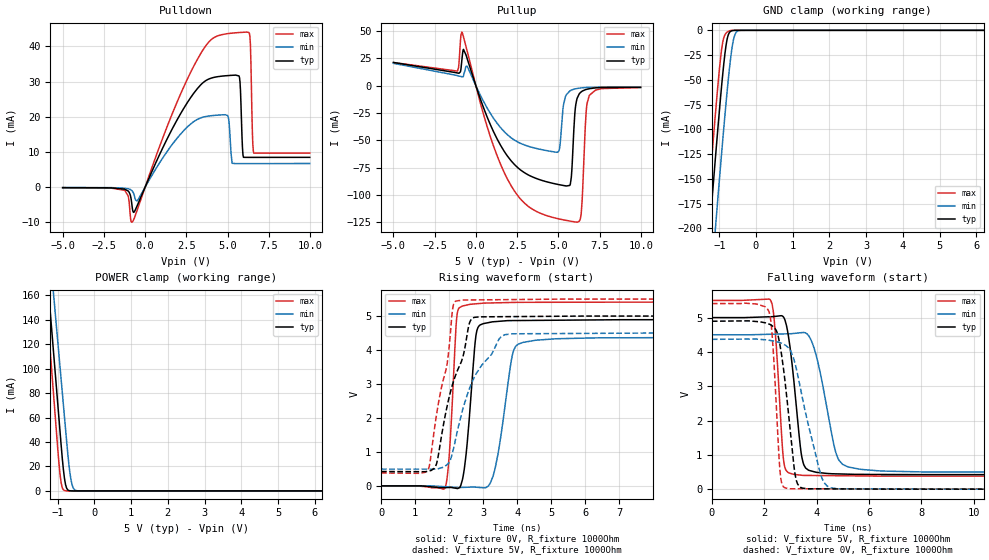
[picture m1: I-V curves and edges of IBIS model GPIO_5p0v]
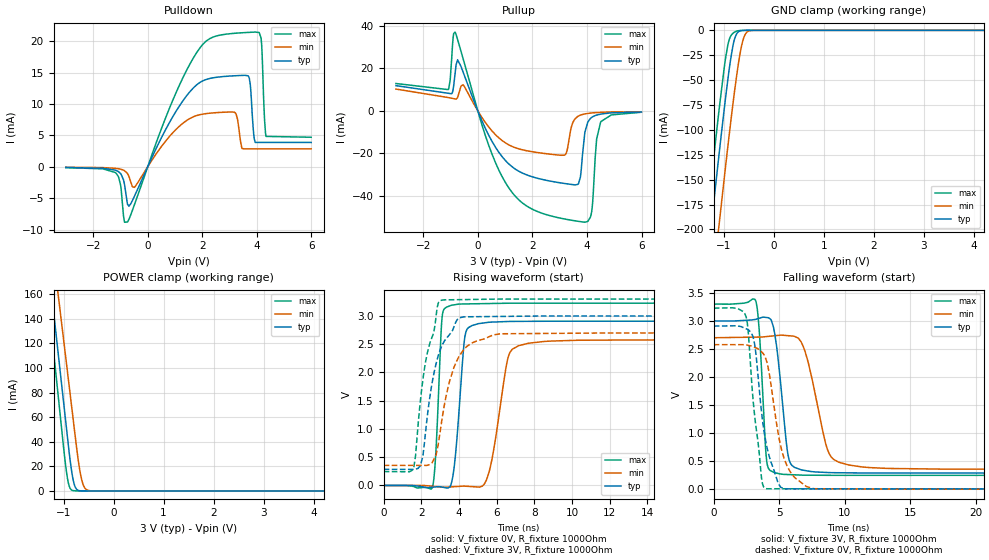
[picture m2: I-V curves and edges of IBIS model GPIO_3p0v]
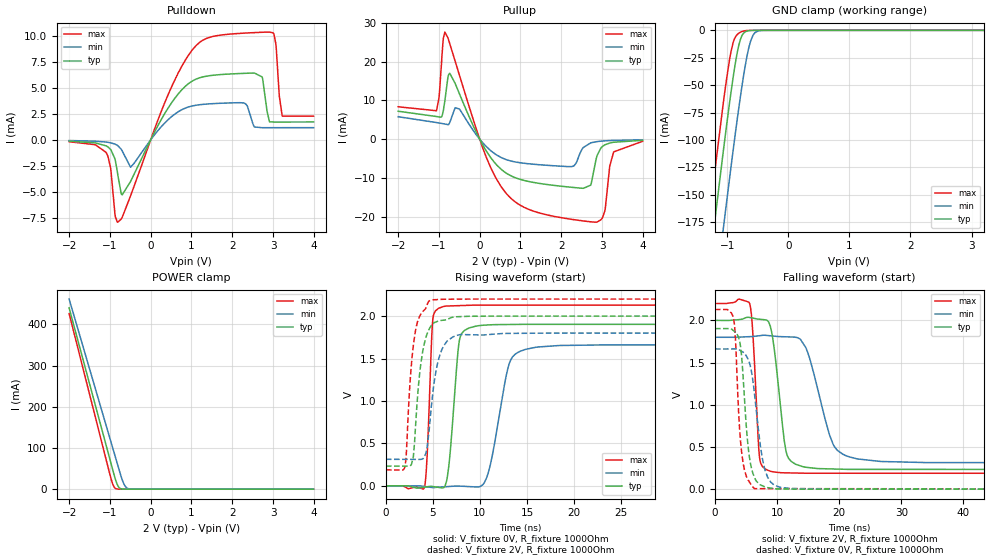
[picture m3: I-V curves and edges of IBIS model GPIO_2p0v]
|Texas Instruments Incorporated
| LMP92018: Analog System Monitor and Controller
| Marketing part#   Digital Voltage Range   Package-type   #pins
| LMP92018   1.8 to 5.5 V   LLP36   36
[IBIS Ver]   4.0
[File name]   lmp92018.ibs
[File Rev]   1.0
[Date]   02/22/2012
[Source]   Texas Instruments Incorporated.
   Analog-eLab, HPA
   12500 TI Blvd
   Dallas, TX -75243
   For Support e-mail: elab_ibis@list.ti.com
[Notes]   Revision History:
   1.0: 02/22/2012
   - Initial version of the model
   - Initial Model generated from simulations
   - Model not matched to measurements
   - Models with trailing _5p0v are generated based on 5.0V
   power supply.
   - Models with trailing _3p0v are generated based on 3.0V
   power supply.
   - Models with trailing _2p0v are generated based on 2.0V
   power supply.
   - C_comp although listed in numerical order of value are
   obtained from varying PVT conditions. For PVT conditions
   for each specific value refer the buffer description under
   respective [Model]. IBIS model user is responsible for using
   appropriate C_comp to simulate for Signal Integrity.
   - Combined pullup/Pulldown non-monotonic warning for DOUT_xxxx and GPIO_xxxx ,is based on
   SPICE simulations and accepted.
[Disclaimer]
  This model is designed as an aid for customers of Texas Instruments.
  TI and its licensors and suppliers make no warranties, either expressed
  or implied, with respect to this model, including the warranties of
  merchantability or fitness for a particular purpose.  The model is
  provided solely on an "as is" basis.  The entire risk as to its quality
  and performance is with the customer.
[Copyright] (C) Copyright 2012 Texas Instruments Incorporated.
   All rights reserved.
|   Device
[Component]   LMP92018
[Manufacturer] TI
[Package]   | 36 pin LLP
| variable   typ   min   max
R_pkg   0.01   0.008   0.12
L_pkg   0.1nH   0.08nH   0.12nH
C_pkg   0.1pF   0.08pF   0.12pF
|-------------------------PIN------------------------------------------------
[Pin] signal_name  model_name  R_pin  L_pin C_pin
1   VDD   POWER   NA   NA   NA
2   GND   GND   NA   NA   NA
3   GND   GND   NA   NA   NA
4   VGPIO   POWER   NA   NA   NA
5   VIO   POWER   NA   NA   NA
6   CSB   DIN   NA   NA   NA
7   SCLK   DIN   NA   NA   NA
8   DIN   DIN   NA   NA   NA
9   DOUT   DOUT   NA   NA   NA
10   OUT3   TERM   NA   NA   NA
11   OUT2   TERM   NA   NA   NA
12   OUT1   TERM   NA   NA   NA
13   OUT0   TERM   NA   NA   NA
14   GND   GND   NA   NA   NA
15   GPIO11   GPIO   NA   NA   NA
16   GPIO10   GPIO   NA   NA   NA
17   GPIO9   GPIO   NA   NA   NA
18   GPIO8   GPIO   NA   NA   NA
19   DRDYB   GPIO   NA   NA   NA
20   GPIO7   GPIO   NA   NA   NA
21   GPIO6   GPIO   NA   NA   NA
22   GPIO5   GPIO   NA   NA   NA
23   GPIO4   GPIO   NA   NA   NA
24   GPIO3   GPIO   NA   NA   NA
25   GPIO2   GPIO   NA   NA   NA
26   GPIO1   GPIO   NA   NA   NA
27   GPIO0   GPIO   NA   NA   NA
28   IN0   TERM   NA   NA   NA
29   IN1   TERM   NA   NA   NA
30   IN2   TERM   NA   NA   NA
31   IN3   TERM   NA   NA   NA
32   IN4   TERM   NA   NA   NA
33   IN5   TERM   NA   NA   NA
34   IN6   TERM   NA   NA   NA
35   IN7   TERM   NA   NA   NA
36   REF   TERM   NA   NA   NA
[Model Selector] GPIO
GPIO_5p0v   model for 5.0v operation
GPIO_3p0v   model for 3.0v operation
GPIO_2p0v   model for 2.0v operation
[Model Selector] DRDYB
DRDYB_5p0v   model for 5.0v operation
DRDYB_3p0v   model for 3.0v operation
DRDYB_2p0v   model for 2.0v operation
[Model Selector] DOUT
DOUT_5p0v   model for 5.0v operation
DOUT_3p0v   model for 3.0v operation
DOUT_2p0v   model for 2.0v operation
[Model Selector] DIN
DIN_5p0v   model for 5.0v operation
DIN_3p0v   model for 3.0v operation
DIN_2p0v   model for 2.0v operation
[Model Selector] TERM
TERM_5p0v   model for 5.0v operation
TERM_3p0v   model for 3.0v operation
TERM_2p0v   model for 2.0v operation
|   Model
[Model] TERM_5p0v
Model_type Terminator
C_comp   1fF   1fF   1fF
| variable   typ   min   max
[Voltage Range]   5.0V   4.5V   5.5V
[POWER Clamp Reference]  3.3V   3.0V   3.6V
[GND Clamp Reference]   0.0V   0.0V   0.0V
|Operating Temperature
[Temperature Range]   27   125   -40
|   Model
[Model] TERM_3p0v
Model_type Terminator
C_comp   1fF   1fF   1fF
| variable   typ   min   max
[Voltage Range]   3.0V   2.7V   3.3V
[POWER Clamp Reference]  3.3V   3.0V   3.6V
[GND Clamp Reference]   0.0V   0.0V   0.0V
|Operating Temperature
[Temperature Range]   27   125   -40
|   Model
[Model] TERM_2p0v
Model_type Terminator
C_comp   1fF   1fF   1fF
| variable   typ   min   max
[Voltage Range]   2.0V   1.8V   2.2V
[POWER Clamp Reference]  2.0V   1.8V   2.2V
[GND Clamp Reference]   0.0V   0.0V   0.0V
|Operating Temperature
[Temperature Range]   27   125   -40
| Models and submodels in the file (15): GPIO_5p0v (I/O), GPIO_3p0v (I/O), GPIO_2p0v (I/O), DRDYB_5p0v (Open_drain), DRDYB_3p0v (Open_drain), DRDYB_2p0v (Open_drain), DOUT_5p0v (3-state), DOUT_3p0v (3-state), DOUT_2p0v (3-state), DIN_5p0v (Input), DIN_3p0v (Input), DIN_2p0v (Input), TERM_5p0v (Terminator), TERM_3p0v (Terminator), TERM_2p0v (Terminator)
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|   Model
[Model]   GPIO_5p0v
Model_type   I/O
Polarity   Non-Inverting
Enable   Active-Low
Vinl = 1.5
Vinh = 3.5
Vmeas = 2.5
Vref = 0
Cref = 1pF
Rref = 1000000
|   typ   min   max
C_comp   0.5484pF   0.5326pF   0.6429pF
[Voltage Range]   5   4.5   5.5
[Temperature Range]   27   125   -40
[Pullup Reference]   5   4.5   5.5
[Pulldown Reference]   0   0   0
[Power Clamp Reference]   5   4.5   5.5
[GND Clamp Reference]   0   0   0
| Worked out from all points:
|   slope of the pulldown table from 0 to 0.75 V, typ, clamps not added: 94.1 ohm
|   slope of the pullup table from 0 to 0.75 V, typ, clamps not added: 24.2 ohm
|   GND clamp passes 1 mA (typ) near -0.69 V on its own axis
|   POWER clamp passes 1 mA (typ) near -0.73 V on its own axis
|   falling waveform, V_fixture 5V, R_fixture 1000Ohm: 20-80 % time 370ps typ, 610ps min, 246ps max; typ from 5 V to 0.423 V
|   rising waveform, V_fixture 0V, R_fixture 1000Ohm: 20-80 % time 234ps typ, 372ps min, 168ps max; typ from 0 V to 4.89 V
|   rising waveform, V_fixture 5V, R_fixture 1000Ohm: 20-80 % time 712ps typ, 915ps min, 503ps max; typ from 0.423 V to 5 V
|   falling waveform, V_fixture 0V, R_fixture 1000Ohm: 20-80 % time 430ps typ, 776ps min, 237ps max; typ from 4.89 V to 0 V
[Pulldown]
|   Voltage   I(typ)   I(min)   I(max)
-5V       -121.4uA   -83.25uA   -139.1uA
-1.235V   -549.3uA   -280uA     -861.8uA
-785mV    -5.531mA   -1.041mA   -9.878mA
2.875V    26.21mA    18.38mA    33.7mA
5.005V    31.7mA     20.36mA    43.62mA
5.275V    31.79mA    6.811mA    43.77mA
5.725V    31.13mA    6.706mA    43.94mA
5.935V    9.185mA    6.705mA    44.01mA
6.325V    8.477mA    6.703mA    43.67mA
6.505V    8.475mA    6.702mA    15.67mA
6.595V    8.474mA    6.702mA    9.674mA
9.985V    8.489mA    6.745mA    9.672mA
[GND Clamp]
|   Voltage   I(typ)   I(min)   I(max)
-5V       -2.033A    -2.096A    -1.993A
-1.355V   -245.5mA   -317.3mA   -200.1mA
-1.295V   -217.2mA   -289mA     -171.8mA
-1.235V   -189mA     -260.8mA   -143.7mA
-1.085V   -120.2mA   -191.3mA   -75.94mA
-965mV    -68.09mA   -137.1mA   -28.27mA
-905mV    -44.2mA    -110.9mA   -11.84mA
-815mV    -15.11mA   -73.28mA   -2.869mA
-725mV    -2.273mA   -39.39mA   -563.2uA
-605mV    -117.9uA   -8.115mA   -20.96uA
-425mV    -723nA     -91.69uA   0A
9.985V    0A         0A         0A
[Pullup]
|   Voltage   I(typ)   I(min)   I(max)
-5V       21.36mA    20.57mA    21.3mA
-1.115V   11.71mA    9.277mA    13.48mA
-845mV    24.37mA    8.276mA    49.16mA
1.495V    -54.47mA   -38.27mA   -71.85mA
3.805V    -85.62mA   -57.83mA   -116mA
5.035V    -90.46mA   -59.55mA   -121.8mA
5.695V    -91.17mA   -4.744mA   -123.8mA
6.115V    -12.72mA   -2.534mA   -124.8mA
6.385V    -5.556mA   -1.941mA   -117.1mA
6.685V    -3.366mA   -1.538mA   -23.79mA
6.865V    -2.715mA   -1.367mA   -9.358mA
9.985V    -1.455mA   -1.278mA   -1.536mA
[POWER Clamp]
|   Voltage   I(typ)   I(min)   I(max)
-5V       1.544A     1.478A     1.599A
-1.415V   225mA      263.7mA    197.8mA
-1.235V   158.9mA    202.9mA    127.5mA
-1.115V   114.8mA    162.3mA    80.59mA
-1.085V   103.8mA    152.2mA    68.87mA
-935mV    48.74mA    101.5mA    13.75mA
-875mV    27.25mA    81.23mA    2.668mA
-815mV    10.54mA    60.97mA    354.1uA
-755mV    2.26mA     40.7mA     71.99uA
-635mV    45.58uA    8.846mA    0A
-485mV    0A         242.3uA    0A
9.985V    0A         0A         0A
[Ramp]
R_load = 1000
|   typ   min   max
dV/dt_r   2.93594/2.33745e-10   2.6197/3.71521e-10   3.24573/1.67105e-10
dV/dt_f   2.7461/3.6989e-10   2.40386/6.10298e-10   3.07209/2.45382e-10
[Falling Waveform]
V_fixture = 5V
V_fixture_min = 4.5V
V_fixture_max = 5.5V
R_fixture = 1000Ohm
C_fixture = 0F
|   Time   V(typ)   V(min)   V(max)
0s        5V         4.5V       5.5V
2.255ns   5.026V     4.515V     5.485V
2.415ns   5.035V     4.518V     4.611V
2.754ns   4.989V     4.525V     750.6mV
2.993ns   4.079V     4.529V     462.5mV
3.442ns   906mV      4.563V     404.2mV
3.9ns     508.1mV    4.11V      398.3mV
4.843ns   444mV      853.7mV    391.6mV
6.348ns   428.5mV    535.4mV    380.9mV
100ns     423.2mV    493.6mV    379.8mV
[Rising Waveform]
V_fixture = 0V
V_fixture_min = 0V
V_fixture_max = 0V
R_fixture = 1000Ohm
C_fixture = 0F
|   Time   V(typ)   V(min)   V(max)
0s        2.277nV    157.5nV    78.77nV
1.879ns   -52.5mV    -25.58mV   -53.48mV
2.217ns   -74.37mV   -46.03mV   4.919V
2.319ns   -32.53mV   -48.12mV   5.257V
2.787ns   4.438V     -39.29mV   5.361V
3.006ns   4.777V     -56.95mV   5.38V
3.351ns   4.836V     525.4mV    5.389V
3.9ns     4.867V     4.008V     5.401V
5.128ns   4.877V     4.33V      5.406V
100ns     4.893V     4.366V     5.41V
[Rising Waveform]
V_fixture = 5V
V_fixture_min = 4.5V
V_fixture_max = 5.5V
R_fixture = 1000Ohm
C_fixture = 0F
|   Time   V(typ)   V(min)   V(max)
0s        423.2mV    493.6mV    379.8mV
1.383ns   433.1mV    493.3mV    481.1mV
1.63ns    652.1mV    493.2mV    2.105V
1.941ns   2.35V      629.2mV    3.601V
2.115ns   3.038V     1.045V     5.294V
2.391ns   3.764V     2.229V     5.471V
2.68ns    4.936V     3.07V      5.474V
3.474ns   4.981V     4.335V     5.482V
3.9ns     4.984V     4.478V     5.486V
100ns     5V         4.5V       5.5V
[Falling Waveform]
|Gnd
V_fixture = 0V
V_fixture_min = 0V
V_fixture_max = 0V
R_fixture = 1000Ohm
C_fixture = 0F
|   Time   V(typ)   V(min)   V(max)
0s        4.893V     4.366V     5.41V
2.173ns   4.813V     4.34V      5.185V
2.337ns   4.74V      4.319V     4.094V
2.62ns    4.102V     4.264V     372mV
2.993ns   1.696V     4.049V     10.82mV
3.177ns   424.5mV    3.653V     10.8mV
3.342ns   74.09mV    3.081V     10.78mV
4.19ns    9.5mV      344.7mV    10.68mV
4.812ns   7.572mV    12.26mV    10.61mV
100ns     2.888uV    5.614uV    1.646uV
|   Model
[Model]   GPIO_3p0v
Model_type   I/O
Polarity   Non-Inverting
Enable   Active-Low
Vinl = 0.9
Vinh = 2.1
Vmeas = 1.5
Vref = 0
Cref = 1pF
Rref = 1000000
|   typ   min   max
C_comp   0.5484pF   0.5326pF   0.6429pF
[Voltage Range]   3   2.7   3.3
[Temperature Range]   27   125   -40
[Pullup Reference]   3   2.7   3.3
[Pulldown Reference]   0   0   0
[Power Clamp Reference]   3   2.7   3.3
[GND Clamp Reference]   0   0   0
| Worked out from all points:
|   slope of the pulldown table from 0 to 0.45 V, typ, clamps not added: 108 ohm
|   slope of the pullup table from 0 to 0.45 V, typ, clamps not added: 35.4 ohm
|   GND clamp passes 1 mA (typ) near -0.69 V on its own axis
|   POWER clamp passes 1 mA (typ) near -0.73 V on its own axis
|   falling waveform, V_fixture 3V, R_fixture 1000Ohm: 20-80 % time 697ps typ, 1.29ns min, 413ps max; typ from 3 V to 0.286 V
|   rising waveform, V_fixture 0V, R_fixture 1000Ohm: 20-80 % time 394ps typ, 703ps min, 251ps max; typ from 0 V to 2.91 V
|   rising waveform, V_fixture 3V, R_fixture 1000Ohm: 20-80 % time 883ps typ, 978ps min, 861ps max; typ from 0.286 V to 3 V
|   falling waveform, V_fixture 0V, R_fixture 1000Ohm: 20-80 % time 984ps typ, 1.19ns min, 766ps max; typ from 2.91 V to 0 V
[Pulldown]
|   Voltage   I(typ)   I(min)   I(max)
-3V       -104.7uA   -65.36uA   -125.4uA
-1.173V   -552.8uA   -244.4uA   -968.2uA
-741mV    -5.952mA   -1.062mA   -8.811mA
-489mV    -4.721mA   -3.272mA   -6.08mA
1.527V    11.88mA    7.662mA    16.23mA
2.913V    14.45mA    8.73mA     21.18mA
3.705V    14.34mA    2.858mA    21.44mA
3.903V    4.476mA    2.858mA    21.48mA
4.083V    3.889mA    2.858mA    21.42mA
4.173V    3.889mA    2.858mA    19.61mA
4.335V    3.888mA    2.859mA    4.851mA
5.991V    3.889mA    2.865mA    4.717mA
[GND Clamp]
|   Voltage   I(typ)   I(min)   I(max)
-3V       -1.048A    -1.117A    -1.005A
-1.353V   -244.6mA   -316.4mA   -199.2mA
-1.335V   -236mA     -307.9mA   -190.7mA
-1.191V   -168.6mA   -240.2mA   -123.4mA
-1.083V   -119.3mA   -190.3mA   -75.08mA
-921mV    -50.35mA   -117.8mA   -15.35mA
-849mV    -24.69mA   -87.18mA   -4.758mA
-777mV    -7.429mA   -58.35mA   -1.564mA
-687mV    -906.9uA   -27.12mA   -224.8uA
-615mV    -152uA     -9.747mA   -28.68uA
-471mV    -2.964uA   -321uA     0A
5.991V    0A         0A         0A
[Pullup]
|   Voltage   I(typ)   I(min)   I(max)
-3V       11.89mA    10.28mA    12.9mA
-1.083V   8.307mA    6.274mA    10.03mA
-831mV    17.82mA    5.623mA    37.15mA
-543mV    18.44mA    12.31mA    24.81mA
1.131V    -24.98mA   -16.01mA   -36.25mA
3.165V    -34.24mA   -20.93mA   -50.97mA
3.687V    -34.4mA    -2.45mA    -52.11mA
3.831V    -21.18mA   -1.72mA    -52.39mA
4.155V    -3.259mA   -1.014mA   -48.67mA
4.353V    -1.99mA    -806.9uA   -13.29mA
4.497V    -1.543mA   -702uA     -5.404mA
5.991V    -555.8uA   -444uA     -662.4uA
[POWER Clamp]
|   Voltage   I(typ)   I(min)   I(max)
-3V       807.8mA    800.2mA    817.2mA
-1.335V   195.7mA    236.7mA    166.5mA
-1.209V   149.4mA    194.1mA    117.3mA
-1.083V   103.1mA    151.5mA    68.09mA
-939mV    50.2mA     102.9mA    14.88mA
-885mV    30.63mA    84.61mA    3.715mA
-831mV    14.28mA    66.37mA    587.4uA
-759mV    2.55mA     42.05mA    79.3uA
-651mV    76.16uA    11.69mA    5.995uA
-597mV    13.99uA    4.084mA    0A
-507mV    0A         434.8uA    0A
5.991V    0A         0A         0A
[Ramp]
R_load = 1000
|   typ   min   max
dV/dt_r   1.74494/3.93131e-10   1.54609/7.03193e-10   1.93662/2.50281e-10
dV/dt_f   1.62821/6.9698e-10   1.40672/1.29096e-09   1.83218/4.1271e-10
[Falling Waveform]
V_fixture = 3V
V_fixture_min = 2.7V
V_fixture_max = 3.3V
R_fixture = 1000Ohm
C_fixture = 0F
|   Time   V(typ)   V(min)   V(max)
0s        3V         2.7V       3.3V
3.195ns   3.028V     2.712V     3.365V
4.044ns   3.061V     2.721V     500.2mV
4.577ns   2.87V      2.734V     301mV
5.112ns   1.877V     2.747V     269.9mV
5.991ns   419.2mV    2.731V     257.6mV
7.001ns   331.4mV    2.435V     249.2mV
8.813ns   295.8mV    634.4mV    247.1mV
11.31ns   288.9mV    396.8mV    246.6mV
100ns     286.3mV    355.5mV    246.4mV
[Rising Waveform]
V_fixture = 0V
V_fixture_min = 0V
V_fixture_max = 0V
R_fixture = 1000Ohm
C_fixture = 0F
|   Time   V(typ)   V(min)   V(max)
0s        41.74nV    93.07nV    97.09nV
2.58ns    -30.66mV   -13.19mV   -42.1mV
3.121ns   -29.83mV   -29.56mV   3.03V
3.617ns   67.81mV    -23.95mV   3.191V
4.006ns   1.348V     -15.87mV   3.212V
4.464ns   2.782V     -15.2mV    3.214V
5.597ns   2.889V     239.9mV    3.221V
6.703ns   2.904V     2.356V     3.227V
8.528ns   2.907V     2.55V      3.228V
100ns     2.908V     2.577V     3.228V
[Rising Waveform]
V_fixture = 3V
V_fixture_min = 2.7V
V_fixture_max = 3.3V
R_fixture = 1000Ohm
C_fixture = 0F
|   Time   V(typ)   V(min)   V(max)
0s        286.3mV    355.5mV    246.4mV
1.6ns     284mV      355.1mV    320mV
1.938ns   343.7mV    355mV      1.461V
2.241ns   997.7mV    354.9mV    2.216V
2.777ns   2.147V     532.8mV    2.981V
3.158ns   2.518V     1.298V     3.285V
3.7ns     2.782V     2.061V     3.288V
4.258ns   2.985V     2.409V     3.291V
6.214ns   2.992V     2.685V     3.3V
100ns     3V         2.7V       3.3V
[Falling Waveform]
|Gnd
V_fixture = 0V
V_fixture_min = 0V
V_fixture_max = 0V
R_fixture = 1000Ohm
C_fixture = 0F
|   Time   V(typ)   V(min)   V(max)
0s        2.908V     2.577V     3.228V
2.473ns   2.86V      2.574V     3.072V
2.64ns    2.843V     2.565V     2.78V
3.114ns   2.596V     2.53V      1.329V
3.683ns   1.306V     2.441V     142.5mV
4.044ns   768.9mV    2.274V     7.422mV
4.921ns   103.5mV    993.9mV    7.354mV
5.462ns   6.061mV    491.9mV    7.312mV
7.629ns   5.922mV    9.148mV    7.144mV
100ns     2.017uV    4.268uV    1.077uV
|   Model
[Model]   GPIO_2p0v
Model_type   I/O
Polarity   Non-Inverting
Enable   Active-Low
Vinl = 0.6
Vinh = 1.4
Vmeas = 1
Vref = 0
Cref = 1pF
Rref = 1000000
|   typ   min   max
C_comp   0.5484pF   0.5326pF   0.6429pF
[Voltage Range]   2   1.8   2.2
[Temperature Range]   27   125   -40
[Pullup Reference]   2   1.8   2.2
[Pulldown Reference]   0   0   0
[Power Clamp Reference]   2   1.8   2.2
[GND Clamp Reference]   0   0   0
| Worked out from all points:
|   slope of the pulldown table from 0 to 0.3 V, typ, clamps not added: 135 ohm
|   slope of the pullup table from 0 to 0.3 V, typ, clamps not added: 58.2 ohm
|   GND clamp passes 1 mA (typ) near -0.69 V on its own axis
|   POWER clamp passes 1 mA (typ) near -0.73 V on its own axis
|   falling waveform, V_fixture 2V, R_fixture 1000Ohm: 20-80 % time 1.56ns typ, 3.19ns min, 821ps max; typ from 2 V to 0.233 V
|   rising waveform, V_fixture 0V, R_fixture 1000Ohm: 20-80 % time 791ps typ, 1.59ns min, 439ps max; typ from 0 V to 1.9 V
|   rising waveform, V_fixture 2V, R_fixture 1000Ohm: 20-80 % time 937ps typ, 1.08ns min, 838ps max; typ from 0.233 V to 2 V
|   falling waveform, V_fixture 0V, R_fixture 1000Ohm: 20-80 % time 1.2ns typ, 1.7ns min, 968ps max; typ from 1.9 V to 0 V
[Pulldown]
|   Voltage   I(typ)   I(min)   I(max)
-2V       -127.3uA   -62.25uA   -178.2uA
-1.094V   -572.8uA   -209.7uA   -1.198mA
-806mV    -3.361mA   -556uA     -7.894mA
-698mV    -5.27mA    -1.063mA   -7.424mA
-494mV    -3.995mA   -2.62mA    -5.378mA
766mV     4.808mA    2.896mA    7.076mA
1.822V    6.29mA     3.526mA    10.1mA
2.734V    6.034mA    1.167mA    10.32mA
2.914V    1.729mA    1.168mA    10.34mA
3.01V     1.713mA    1.168mA    10.23mA
3.226V    1.713mA    1.169mA    2.278mA
3.994V    1.714mA    1.171mA    2.274mA
[GND Clamp]
|   Voltage   I(typ)   I(min)   I(max)
-2V       -557mA     -627.9mA   -512.6mA
-1.562V   -344.5mA   -416.1mA   -299.3mA
-1.262V   -201.7mA   -273.5mA   -156.3mA
-1.238V   -190.4mA   -262.2mA   -145.1mA
-1.058V   -108.2mA   -178.9mA   -64.38mA
-962mV    -66.85mA   -135.8mA   -27.27mA
-902mV    -43.08mA   -109.6mA   -11.26mA
-782mV    -8.241mA   -60.27mA   -1.702mA
-638mV    -271.3uA   -14.28mA   -57.64uA
-566mV    -42.51uA   -3.593mA   -5.697uA
-482mV    -4.099uA   -431.6uA   0A
3.994V    0A         0A         0A
[Pullup]
|   Voltage   I(typ)   I(min)   I(max)
-2V       7.195mA    5.781mA    8.341mA
-1.058V   5.826mA    4.273mA    7.319mA
-854mV    9.869mA    3.893mA    27.58mA
-734mV    16.98mA    4.274mA    24.62mA
-494mV    11.61mA    7.75mA     16.4mA
526mV     -7.752mA   -4.722mA   -12.22mA
2.314V    -12.46mA   -6.851mA   -20.75mA
2.722V    -11.86mA   -971.1uA   -21.3mA
2.986V    -2.123mA   -509.1uA   -20.62mA
3.07V     -1.47mA    -440.2uA   -18.5mA
3.286V    -796.8uA   -325.3uA   -3.281mA
3.994V    -308.4uA   -173.6uA   -559.8uA
[POWER Clamp]
|   Voltage   I(typ)   I(min)   I(max)
-2V       440.1mA    461.6mA    426.3mA
-1.01V    76.28mA    126.8mA    39.59mA
-950mV    54.24mA    106.6mA    18.16mA
-914mV    41.02mA    94.41mA    8.567mA
-878mV    28.25mA    82.25mA    2.95mA
-830mV    14.03mA    66.03mA    568.4uA
-794mV    6.602mA    53.87mA    193.6uA
-746mV    1.712mA    37.66mA    58.04uA
-674mV    161.5uA    16.67mA    10.53uA
-590mV    11.32uA    3.49mA     0A
-410mV    0A         32.33uA    0A
3.994V    0A         0A         0A
[Ramp]
R_load = 1000
|   typ   min   max
dV/dt_r   1.14153/7.91251e-10   0.996659/1.59088e-09   1.27753/4.39451e-10
dV/dt_f   1.05992/1.5645e-09   0.892217/3.17962e-09   1.20702/8.20887e-10
[Falling Waveform]
V_fixture = 2V
V_fixture_min = 1.8V
V_fixture_max = 2.2V
R_fixture = 1000Ohm
C_fixture = 0F
|   Time   V(typ)   V(min)   V(max)
0s        2V         1.8V       2.2V
5.613ns   2.034V     1.808V     2.194V
6.144ns   2.026V     1.809V     1.802V
7.182ns   2.013V     1.818V     379.1mV
8.929ns   1.926V     1.818V     212.5mV
11.44ns   449mV      1.805V     193.4mV
14.09ns   267.8mV    1.738V     189.7mV
19.02ns   239.2mV    531.9mV    188.6mV
22.78ns   234.6mV    360.9mV    188.6mV
100ns     233.5mV    313mV      188.3mV
[Rising Waveform]
V_fixture = 0V
V_fixture_min = 0V
V_fixture_max = 0V
R_fixture = 1000Ohm
C_fixture = 0F
|   Time   V(typ)   V(min)   V(max)
0s        9.415nV    87.66nV    6.679nV
4.087ns   -15.24mV   -6.915mV   -21.72mV
4.995ns   -7.608mV   -20.35mV   1.966V
6.144ns   -20.19mV   -11.56mV   2.113V
7.818ns   1.715V     -2.529mV   2.123V
9.587ns   1.882V     -12.54mV   2.129V
10.98ns   1.896V     190.9mV    2.129V
13.29ns   1.901V     1.488V     2.129V
15.86ns   1.902V     1.631V     2.129V
100ns     1.903V     1.661V     2.129V
[Rising Waveform]
V_fixture = 2V
V_fixture_min = 1.8V
V_fixture_max = 2.2V
R_fixture = 1000Ohm
C_fixture = 0F
|   Time   V(typ)   V(min)   V(max)
0s        233.5mV    313mV      188.3mV
2.063ns   232.7mV    312.1mV    243.7mV
2.731ns   257.5mV    311.8mV    1.452V
2.92ns    345mV      311.7mV    1.653V
3.713ns   1.437V     311.6mV    2.021V
4.405ns   1.797V     466.2mV    2.139V
4.842ns   1.889V     943.9mV    2.189V
5.984ns   1.95V      1.613V     2.197V
8.017ns   1.994V     1.782V     2.199V
100ns     2V         1.8V       2.2V
[Falling Waveform]
|Gnd
V_fixture = 0V
V_fixture_min = 0V
V_fixture_max = 0V
R_fixture = 1000Ohm
C_fixture = 0F
|   Time   V(typ)   V(min)   V(max)
0s        1.903V     1.661V     2.129V
2.996ns   1.879V     1.662V     2.022V
3.32ns    1.86V      1.662V     1.764V
3.88ns    1.781V     1.653V     828.4mV
4.494ns   1.382V     1.625V     332.8mV
5.403ns   464mV      1.53V      102.6mV
6.361ns   142.6mV    1.133V     6.435mV
8.017ns   27.99mV    238.3mV    6.321mV
10.7ns    2.487mV    19.53mV    6.137mV
100ns     1.651uV    3.86uV     743nV
